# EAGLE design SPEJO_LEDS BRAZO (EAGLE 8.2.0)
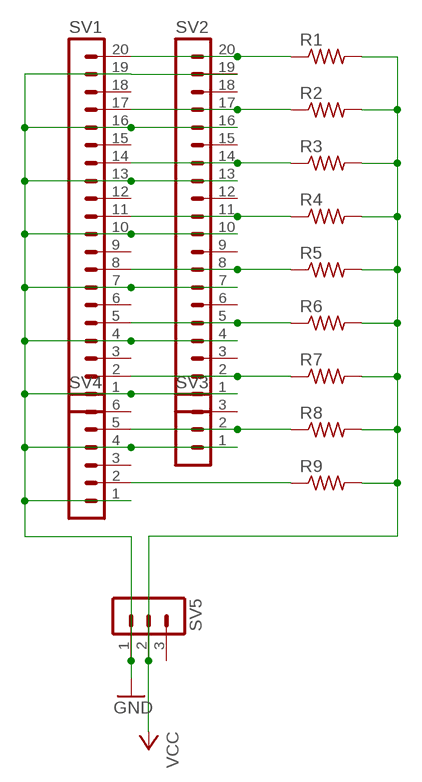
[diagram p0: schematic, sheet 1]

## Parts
R1  RES-US1206FAB  [R1206FAB]
R2  RES-US1206FAB  [R1206FAB]
R3  RES-US1206FAB  [R1206FAB]
R4  RES-US1206FAB  [R1206FAB]
R5  RES-US1206FAB  [R1206FAB]
R6  RES-US1206FAB  [R1206FAB]
R7  RES-US1206FAB  [R1206FAB]
R8  RES-US1206FAB  [R1206FAB]
R9  RES-US1206FAB  [R1206FAB]
SV1  MA20-1  [MA20-1]
SV2  MA20-1  [MA20-1]
SV3  MA03-1  [MA03-1]
SV4  MA06-1  [MA06-1]
SV5  MA03-1  [MA03-1]

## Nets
GND: SV1.1 SV1.4 SV1.7 SV1.10 SV1.13 SV1.16 SV1.19 SV2.1 SV2.4 SV2.7 SV2.10 SV2.13 SV2.16 SV2.19 SV3.1 SV4.1 SV4.4 SV5.1
N$3: R1.1 SV1.20 SV2.20
N$4: R2.1 SV1.17 SV2.17
N$6: R3.1 SV1.14 SV2.14
N$8: R4.1 SV1.11 SV2.11
N$10: R5.1 SV1.8 SV2.8
N$12: R6.1 SV1.5 SV2.5
N$14: R7.1 SV1.2 SV2.2
N$16: R8.1 SV3.2 SV4.5
N$18: R9.1 SV4.2
VCC: R1.2 R2.2 R3.2 R4.2 R5.2 R6.2 R7.2 R8.2 R9.2 SV5.2
Unconnected: SV1.3 SV1.6 SV1.9 SV1.12 SV1.15 SV1.18 SV2.3 SV2.6 SV2.9 SV2.12 SV2.15 SV2.18 SV3.3 SV4.3 SV4.6 SV5.3

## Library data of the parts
R1-R9 = fab:RES-US: Resistor (US Symbol)
SV1 SV2 = con-lstb:MA20-1: PIN HEADER; OC_FARNELL: unknown; OC_NEWARK: unknown
SV3 SV5 = con-lstb:MA03-1: PIN HEADER; OC_FARNELL: unknown; OC_NEWARK: unknown
SV4 = con-lstb:MA06-1: PIN HEADER; OC_FARNELL: unknown; OC_NEWARK: unknown

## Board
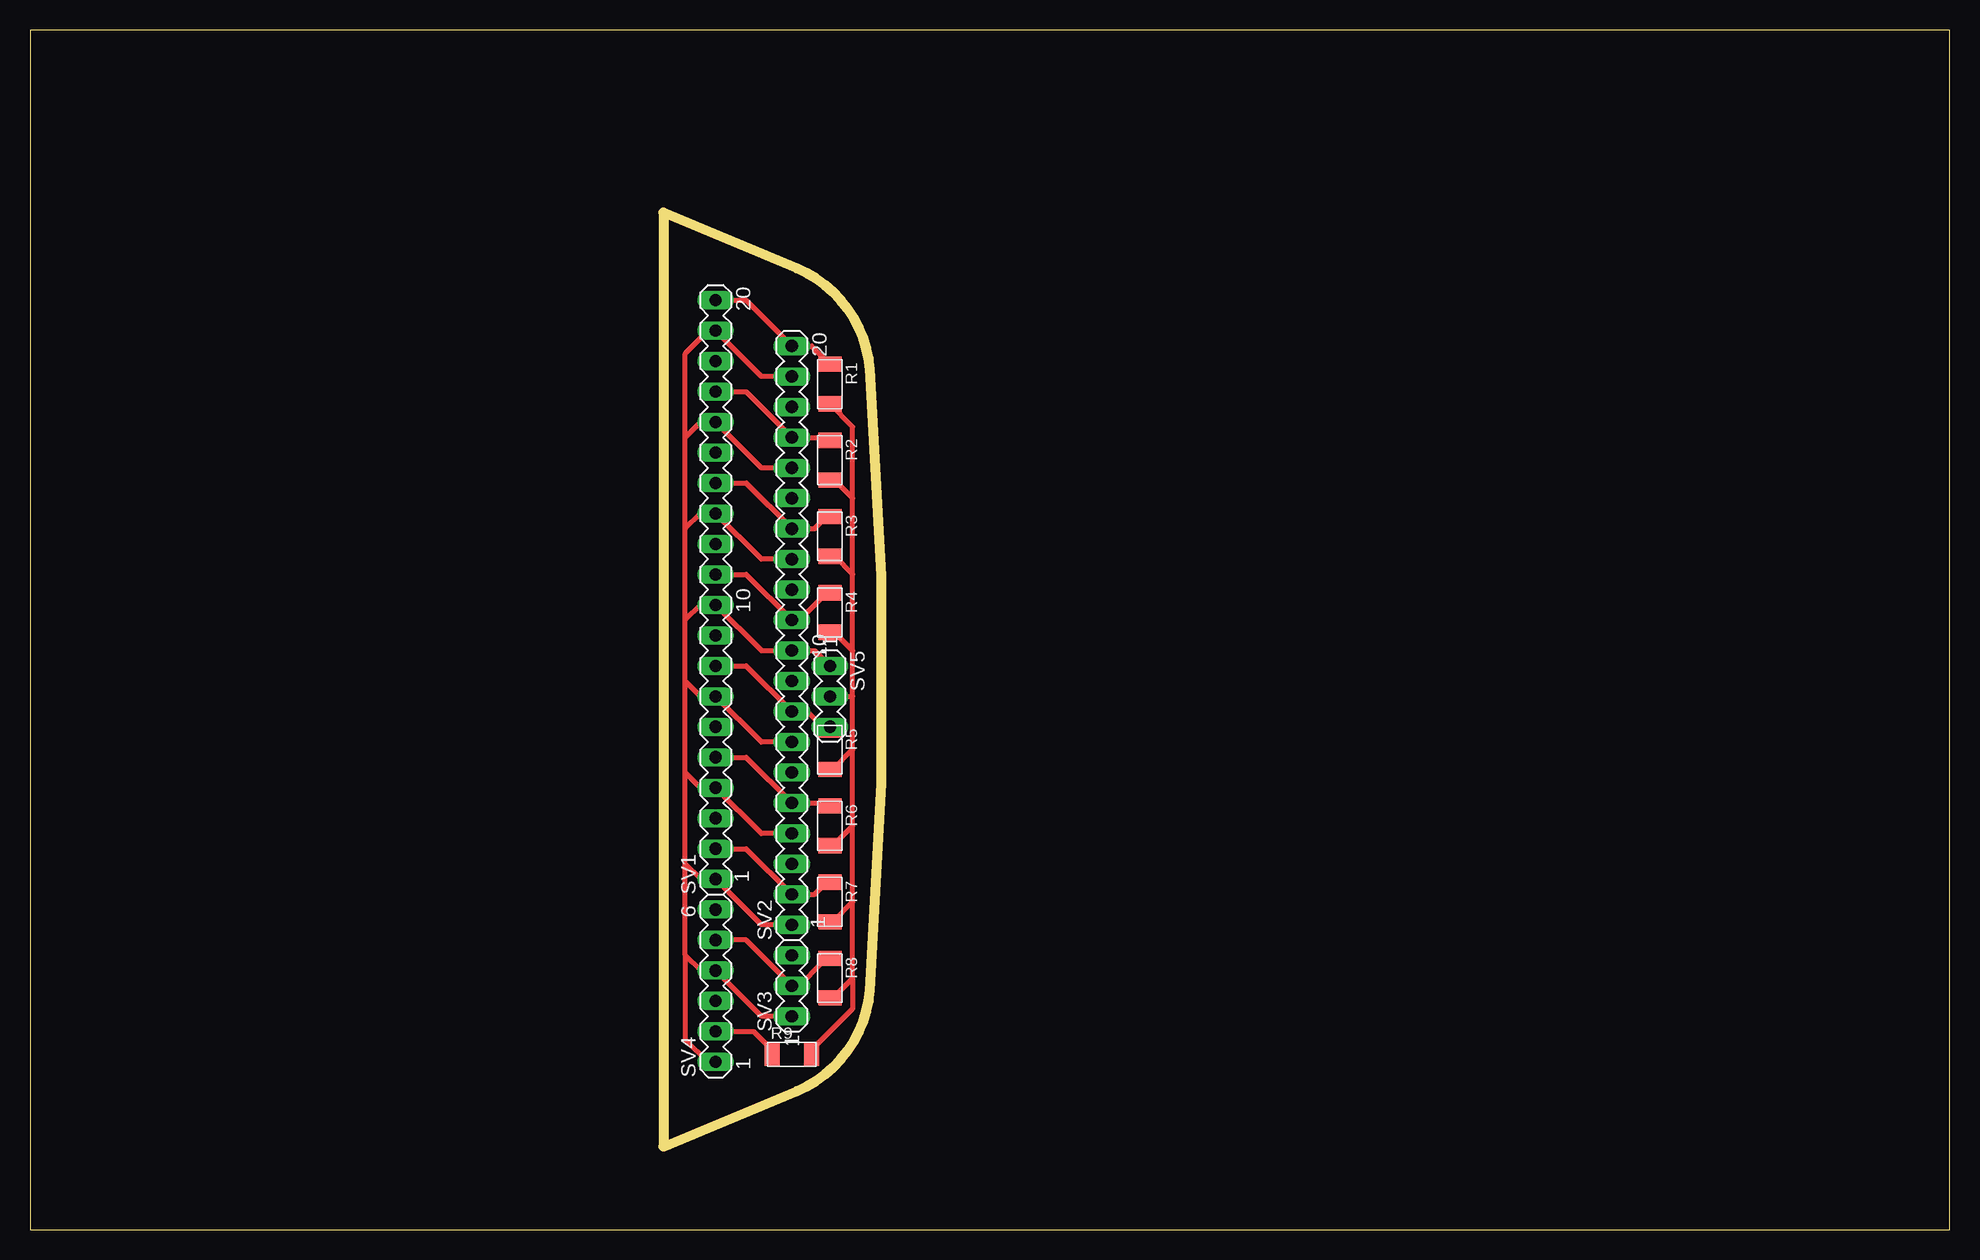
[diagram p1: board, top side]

Size 160 x 100 mm. Coordinates in mm from the lower left corner, seen from the top.
Outline: 0,0 160,0 160,100 0,100 0,0
Outline: 63.91,11.54 arc63 70.02,19.94 arc9 70.02,71.73 arc63 63.91,80.13 52.81,84.77 52.81,6.9 63.91,11.54
Copper layers (1*16): Top 0.035mm / dielectric 1.5mm / Bottom 0.035mm
Design rules "default": minimum track width 6mil, minimum drill 0.35mm, track to track 6mil, track to pad 6mil, pad to pad 6mil, via to via 6mil, smd to smd 6mil, copper to edge 40mil, drill to drill 6mil, minimum pad ring 10mil, minimum via ring 8mil, stop-mask expansion 4mil, vias tented up to drill 0mil, thermal gap 10mil

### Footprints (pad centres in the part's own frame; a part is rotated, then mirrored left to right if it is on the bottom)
R1206FAB = smd 1.27 x 1.905: 1 -1.651,0; 2 1.651,0
MA20-1 = drill 1.016 long: 1 -24.13,0; 2 -21.59,0; 3 -19.05,0; 4 -16.51,0; 5 -13.97,0; 6 -11.43,0; 7 -8.89,0; 8 -6.35,0; 9 -3.81,0; 10 -1.27,0; 11 1.27,0; 12 3.81,0; 13 6.35,0; 14 8.89,0; 15 11.43,0; 16 13.97,0; 17 16.51,0; 18 19.05,0; 19 21.59,0; 20 24.13,0
MA03-1 = drill 1.016 long: 1 -2.54,0; 2 0,0; 3 2.54,0
MA06-1 = drill 1.016 long: 1 -6.35,0; 2 -3.81,0; 3 -1.27,0; 4 1.27,0; 5 3.81,0; 6 6.35,0

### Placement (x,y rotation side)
R1  66.67,70.48 270 top
R2  66.67,64.14 270 top
R3  66.67,57.78 270 top
R4  66.67,51.44 270 top
R5  66.67,40.01 270 top
R6  66.67,33.66 270 top
R7  66.67,27.3 270 top
R8  66.67,20.95 270 top
R9  63.5,14.61 0 top
SV1  57.15,53.34 90 top
SV2  63.5,49.53 90 top
SV3  63.5,20.32 90 top
SV4  57.15,20.32 90 top
SV5  66.67,44.45 270 top

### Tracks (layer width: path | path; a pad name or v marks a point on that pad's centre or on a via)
GND
  Top 0.406: SV2.19 60.96,71.12 SV1.19 56.52,74.93 54.61,73.03 54.61,66.04 | SV2.16 60.96,63.5 SV1.16 55.88,67.31 54.61,66.04 | SV2.13 60.96,55.88 SV1.13 55.88,59.69 54.61,58.42 | SV2.7 60.96,40.64 SV1.7 55.88,44.45 54.61,45.72 | SV2.4 60.96,33.02 SV1.4 55.88,36.83 54.61,38.1 | SV2.1 60.96,25.4 SV1.1 55.88,29.21 54.61,30.48 | SV3.1 60.96,17.78 SV4.4 55.88,21.59 54.61,22.86 | 54.61,58.42 54.61,66.04 | 54.61,50.8 54.61,58.42 | 54.61,45.72 54.61,50.8 | 54.61,38.1 54.61,45.72 | 54.61,30.48 54.61,38.1 | 54.61,22.86 54.61,30.48 | 54.61,22.86 54.61,15.88 56.52,13.97 SV4.1 | 54.61,50.8 55.88,52.07 SV1.10 60.96,48.26 SV2.10 65.41,48.26 SV5.1
N$3
  Top 0.406: SV1.20 59.69,77.47 SV2.20 65.15,73.66 R1.1
N$4
  Top 0.152: 66.42,66.04 R2.1
  Top 0.406: SV1.17 59.69,69.85 SV2.17 66.42,66.04
N$6
  Top 0.152: 66.04,59.05 66.29,59.05 R3.1
  Top 0.406: SV1.14 59.69,62.23 SV2.14 65.41,58.42 66.04,59.05
N$8
  Top 0.152: 66.04,52.7 66.29,52.7 R4.1
  Top 0.406: SV1.11 59.69,54.61 SV2.11 64.14,50.8 66.04,52.7
N$10
  Top 0.152: 66.04,41.91 66.42,41.91 R5.1
  Top 0.406: SV1.8 59.69,46.99 SV2.8 64.77,43.18 66.04,41.91
N$12
  Top 0.152: 66.42,35.56 R6.1
  Top 0.406: SV1.5 59.69,39.37 SV2.5 66.42,35.56
N$14
  Top 0.152: 66.04,28.57 66.29,28.57 R7.1
  Top 0.406: SV1.2 59.69,31.75 SV2.2 65.41,27.94 66.04,28.57
N$16
  Top 0.152: 66.04,22.23 66.29,22.23 R8.1
  Top 0.406: SV4.5 59.69,24.13 SV3.2 64.14,20.32 66.04,22.23
N$18
  Top 0.152: 61.59,15.24 61.59,14.86 R9.1
  Top 0.406: SV4.2 60.33,16.51 61.59,15.24
VCC
  Top 0.152: R9.2 65.15,14.99 | R2.2 67.06,62.48 | R3.2 67.06,56.13 | R4.2 67.06,49.78 | R5.2 66.93,38.35 | R6.2 66.93,32 | R7.2 66.93,25.65 | R8.2 66.93,19.3
  Top 0.406: 65.15,14.99 68.58,18.41 68.58,20.95 | 68.58,54.61 68.58,60.96 | 68.58,48.26 68.58,54.61 | 68.58,44.45 68.58,48.26 | 68.58,40.01 68.58,44.45 | 68.58,33.66 68.58,40.01 | 68.58,27.3 68.58,33.66 | 68.58,20.95 68.58,27.3 | 68.58,60.96 68.58,66.93 R1.2 | 67.06,62.48 68.58,60.96 | 67.06,56.13 68.58,54.61 | 67.06,49.78 68.58,48.26 | SV5.2 68.58,44.45 | 66.93,38.35 68.58,40.01 | 66.93,32 68.58,33.66 | 66.93,25.65 68.58,27.3 | 66.93,19.3 68.58,20.95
